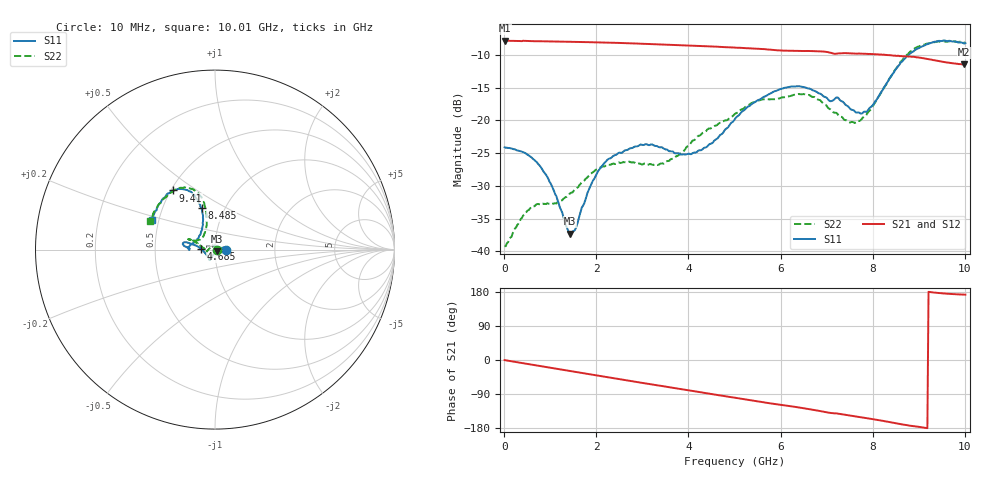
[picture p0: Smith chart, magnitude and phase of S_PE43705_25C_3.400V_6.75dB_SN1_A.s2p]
! Device ID: PE43705
! Serial: 1
! Insertion: A
! Impedance: 50 ohm
! Temp: 25C
! VDD: 3.400V
! Attenuation Step: 6.75dB
#  Hz  S  RI  R  50
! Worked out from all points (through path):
!   401 points, 10 MHz to 10.01 GHz, reference 50 ohm
!   highest |S21| = -7.80 dB at 10 MHz (marker M1); lowest = -11.4 dB at 9.985 GHz (marker M2)
!   group delay of S21, straight-line fit = 53.5 ps
!   lowest |S11| = -37.3 dB at 1.435 GHz (marker M3), VSWR 1.03, Z = 51 - j0.951 ohm
!   |S11| at or under -10 dB: start of sweep to 8.776 GHz
!   |S22| runs from -39.2 to -7.9 dB; largest |S21 - S12| = 0.0038
!   S11 on the Smith chart (normalised r, x): 10 MHz: 1.13, -0.00; 4.685 GHz: 0.86, +0.00; 8.485 GHz: 0.78, +0.38; 9.41 GHz: 0.51, +0.40; 10.01 GHz: 0.46, +0.18
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1e7  0.0623 -0.000156  0.4074 -0.00192  0.4079 -0.00186  0.011 0.00027
4.6e8  0.0552 0.0107  0.3992 -0.0673  0.3993 -0.0665  0.008 0.0181
7.6e8  0.0441 0.0117  0.3881 -0.1082  0.388 -0.1081  -0.000224 0.0229
1.435e9  0.00999 -0.00932  0.3485 -0.1945  0.3488 -0.1943  -0.0251 0.012
1.685e9  -0.00207 -0.0215  0.3289 -0.2232  0.3289 -0.2231  -0.0334 0.00377
1.96e9  -0.0129 -0.0336  0.3045 -0.2525  0.3045 -0.2522  -0.0408 -0.00448
2.235e9  -0.0198 -0.0457  0.2774 -0.279  0.2774 -0.2789  -0.0446 -0.0113
2.935e9  -0.0295 -0.0575  0.1983 -0.3318  0.1988 -0.3319  -0.0456 -0.0107
3.36e9  -0.0311 -0.0543  0.1463 -0.3522  0.1468 -0.3519  -0.0452 -0.0081
4.035e9  -0.0473 -0.0285  0.0605 -0.3684  0.061 -0.3682  -0.0651 0.00998
4.685e9  -0.0772 0.00283  -0.0218 -0.3637  -0.0212 -0.3639  -0.0913 0.0294
5.01e9  -0.1007 0.0203  -0.0603 -0.355  -0.06 -0.3553  -0.1052 0.0393
5.96e9  -0.1667 0.0414  -0.1584 -0.3047  -0.1575 -0.3048  -0.1351 0.0584
6.685e9  -0.1699 0.019  -0.2226 -0.2555  -0.2225 -0.255  -0.1407 0.0565
7.635e9  -0.1027 0.0514  -0.2785 -0.1666  -0.2779 -0.167  -0.0665 0.07
7.91e9  -0.0793 0.0926  -0.2903 -0.1391  -0.2903 -0.1408  -0.0551 0.103
8.36e9  -0.0681 0.1968  -0.3028 -0.0887  -0.3023 -0.0901  -0.0483 0.2027
8.485e9  -0.0751 0.2303  -0.3043 -0.073  -0.3039 -0.0746  -0.0556 0.2379
8.91e9  -0.1294 0.3185  -0.3044 -0.0268  -0.3027 -0.0279  -0.1202 0.3345
9.41e9  -0.2332 0.3293  -0.2851 0.0152  -0.2841 0.0151  -0.2259 0.3327
9.985e9  -0.3458 0.1732  -0.2656 0.0347  -0.2665 0.0345  -0.3533 0.1716
1.001e10  -0.3531 0.164  -0.2664 0.0352  -0.2675 0.0344  -0.3612 0.1604
